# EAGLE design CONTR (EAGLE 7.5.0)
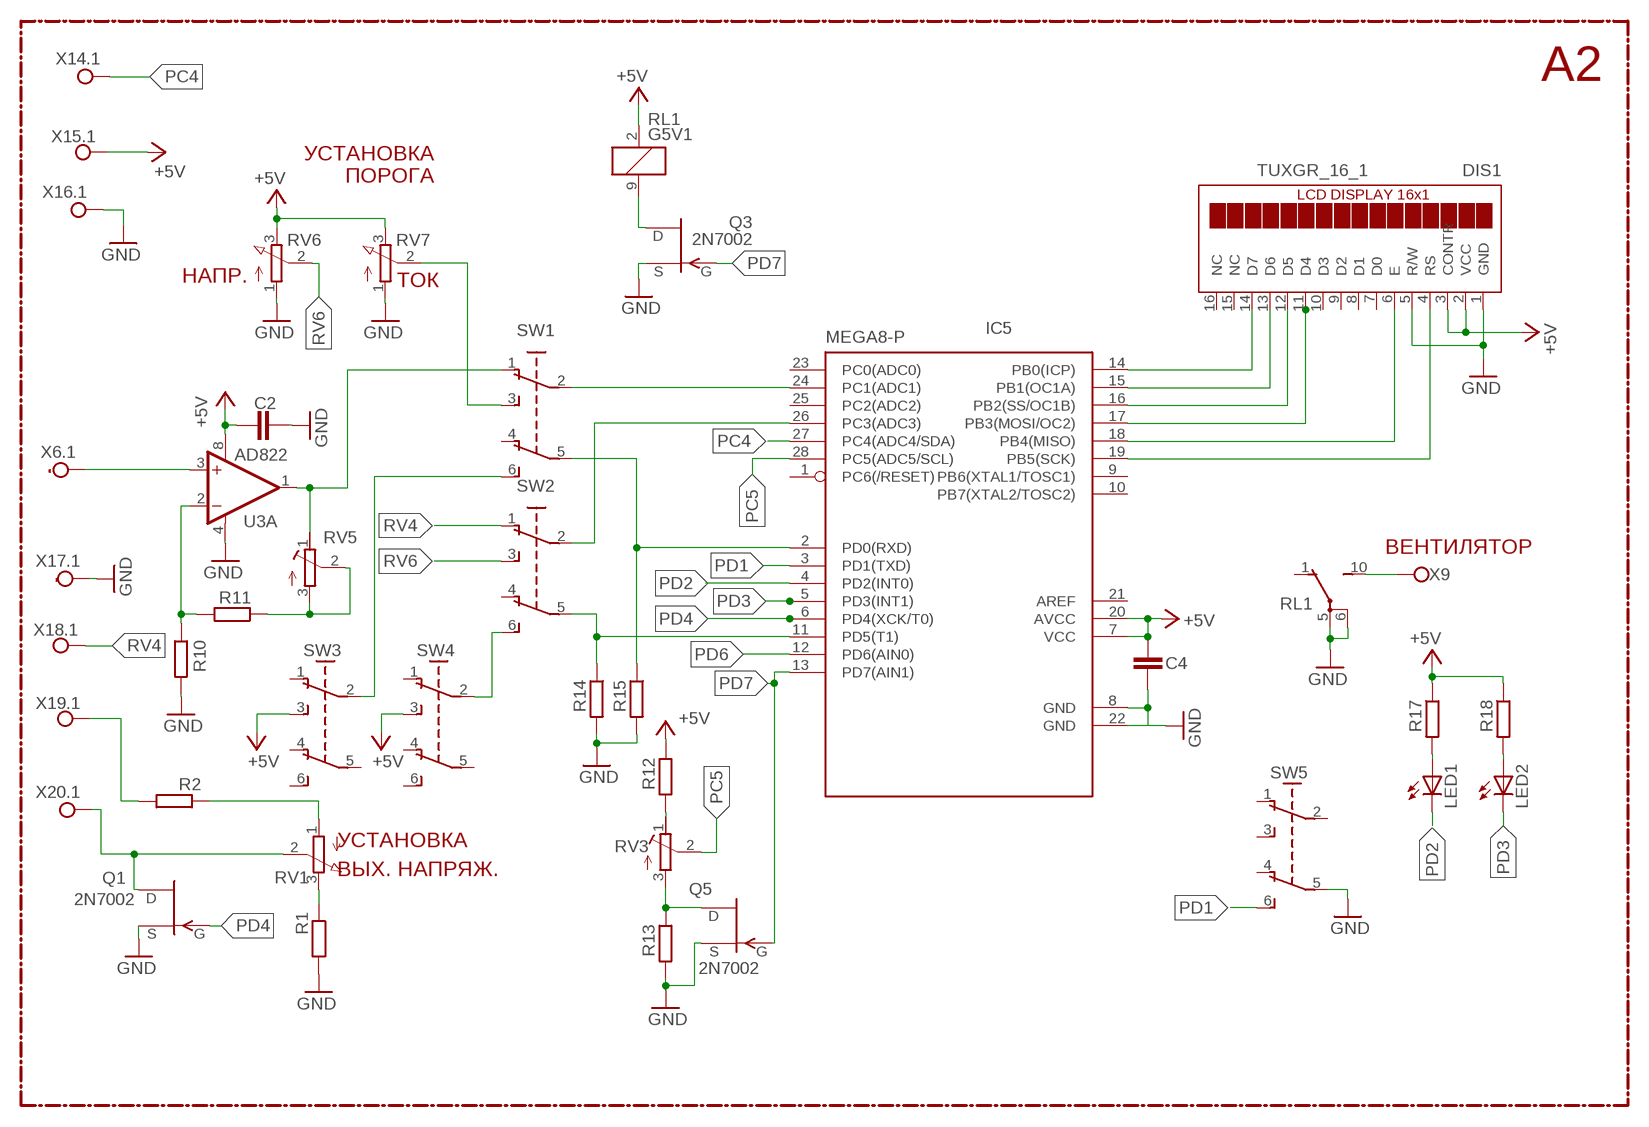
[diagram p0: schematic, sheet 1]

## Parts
C2  C-EUC1206  [C1206]
C4  C-EUC1206  [C1206]
DIS1  TUXGR_16_1  [TUXGR_16X1]
IC5  MEGA8-P  [DIL28-3]
LED1  LED3MM  [LED3MM]
LED2  LED3MM  [LED3MM]
Q1  2N7002  SST201  [SOT23]
Q3  2N7002  SST201  [SOT23]
Q5  2N7002  SST201  [SOT23]
R1  R-EU_R1206  [R1206]
R2  R-EU_R1206  [R1206]
R10  R-EU_R1206  [R1206]
R11  R-EU_R1206  [R1206]
R12  R-EU_R1206  [R1206]
R13  R-EU_R1206  [R1206]
R14  R-EU_R1206  [R1206]
R15  R-EU_R1206  [R1206]
R17  R-EU_R1206  [R1206]
R18  R-EU_R1206  [R1206]
RL1  G5V1  [G5V1]
RV1  PTV09A  PV09A  [PTV09]
RV3  R-TRIMM-3386-F  [R-TRIMM-3386F]
RV5  R-TRIMM-3386-F  [R-TRIMM-3386F]
RV6  PTV09A  PV09A  [PTV09]
RV7  PTV09A  PV09A  [PTV09]
SW1  ESB30B102  [ESB30B102]
SW2  ESB30B102  [ESB30B102]
SW3  ESB30B102  [ESB30B102]
SW4  ESB30B102  [ESB30B102]
SW5  ESB30B102  [ESB30B102]
U3  AD822  OPA2134P  [DIL08]
X6.1  TPPAD1-20  [P1-20]
X9  TPPAD1-20  [P1-20]
X14.1  TPPAD1-20  [P1-20]
X15.1  TPPAD1-20  [P1-20]
X16.1  TPPAD1-20  [P1-20]
X17.1  TPPAD1-20  [P1-20]
X18.1  TPPAD1-20  [P1-20]
X19.1  TPPAD1-20  [P1-20]
X20.1  TPPAD1-20  [P1-20]

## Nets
+5V: C2.2 C4.2 DIS1.2(VCC) DIS1.3(CONTR) IC5.7(VCC) IC5.20(AVCC) R12.1 R17.1 R18.1 RL1.2 RV6.3(E) RV7.3(E) SW3.3 SW4.3 U3.8(A:V+) X15.1.TP
GND: C2.1 C4.1 DIS1.1(GND) DIS1.5(R/W) IC5.8(GND) IC5.22(GND) Q1.2(S) Q3.2(S) Q5.2(S) R1.2 R10.2 R13.2 R14.2 R15.2 RL1.5(2:P) RL1.6(2:P) RV6.1(A) RV7.1(A) SW5.5 U3.4(A:V-) X16.1.TP X17.1.TP
N$2: R2.1 RV1.1(A)
N$3: Q1.1(D) RV1.2(S) X20.1.TP
N$4: R1.1 RV1.3(E)
N$8: U3.3(A:+IN) X6.1.TP
N$14: DIS1.14(D7) IC5.14(PB0(ICP))
N$15: DIS1.13(D6) IC5.15(PB1(OC1A))
N$16: DIS1.12(D5) IC5.16(PB2(SS/OC1B))
N$17: DIS1.11(D4) IC5.17(PB3(MOSI/OC2))
N$18: DIS1.6(E) IC5.18(PB4(MISO))
N$19: DIS1.4(RS) IC5.19(PB5(SCK))
N$20: R10.1 R11.2 U3.2(A:-IN)
N$21: R11.1 RV5.2(S) RV5.3(E)
N$22: IC5.24(PC1(ADC1)) SW1.2
N$23: RV7.2(S) SW1.3
N$24: RV5.1(A) SW1.1 U3.1(A:OUT)
N$25: Q3.1(D) RL1.9
N$26: SW1.6 SW3.2
N$27: IC5.26(PC3(ADC3)) SW2.2
N$29: IC5.11(PD5(T1)) R14.1 SW2.5
N$30: SW2.6 SW4.2
N$31: IC5.2(PD0(RXD)) R15.1 SW1.5
N$32: RL1.10(2:S) X9.TP
N$35: R12.2 RV3.1(A)
N$36: Q5.1(D) R13.1 RV3.3(E)
N$39: R2.2 X19.1.TP
N$40: LED2.A R18.2
N$41: LED1.A R17.2
PC4: IC5.27(PC4(ADC4/SDA)) X14.1.TP
PC5: IC5.28(PC5(ADC5/SCL)) RV3.2(S)
PD1: IC5.3(PD1(TXD)) SW5.6
PD2: IC5.4(PD2(INT0)) LED1.K(C)
PD3: IC5.5(PD3(INT1)) LED2.K(C)
PD4: IC5.6(PD4(XCK/T0)) Q1.3(G)
PD6: IC5.12(PD6(AIN0))
PD7: IC5.13(PD7(AIN1)) Q3.3(G) Q5.3(G)
RV4: SW2.1 X18.1.TP
RV6: RV6.2(S) SW2.3
Unconnected: DIS1.7(D0) DIS1.8(D1) DIS1.9(D2) DIS1.10(D3) DIS1.15(NC) DIS1.16(NC) IC5.1(PC6(/RESET)) IC5.9(PB6(XTAL1/TOSC1)) IC5.10(PB7(XTAL2/TOSC2)) IC5.21(AREF) IC5.23(PC0(ADC0)) IC5.25(PC2(ADC2)) RL1.1(2:O) SW1.4 SW2.4 SW3.1 SW3.4 SW3.5 SW3.6 SW4.1 SW4.4 SW4.5 SW4.6 SW5.1 SW5.2 SW5.3 SW5.4 U3.5(B:+IN) U3.6(B:-IN) U3.7(B:OUT)

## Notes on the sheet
- A2
- УСТАНОВКА
- ПОРОГА
- НАПР. | ТОК
- ВЕНТИЛЯТОР
- УСТАНОВКА
- ВЫХ. НАПРЯЖ.

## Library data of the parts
C2 C4 = rcl:C-EU: CAPACITOR, European symbol
DIS1 = display-lcd:TUXGR_16_1: 1x16 LCD DISPLAY
IC5 = atmel:MEGA8-P: MICROCONTROLLER 8 Kbytes FLASH, 1 kbytes SRAM, 512 bytes EEPROM, USART, 4-channel 10 bit ADC, 2-channel 8 bit ADC Pin compatible with Atmega48, ATMega88, ATMega168 Source: avr.lbr; OC_FARNELL: unknown; OC_NEWARK: unknown
LED1 LED2 = led:LED: LED
Q1 Q3 Q5 = transistor-fet:?20*: TEMIC / Siliconix N-Channel JFET Source: JFET-J201_Siliconix_data.pdf
R1 R2 R10-R15 R17 R18 = rcl:R-EU_: RESISTOR, European symbol
RL1 = relay:G5V1: RELAY 1 x switch, 0.5 A/125 V AC, 1 A/24 V DC , Omron; MPN: G5V-1-DC24; OC_FARNELL: 9949593; OC_NEWARK: 36M6377
RV1 RV6 RV7 = pot:PV09A
RV3 RV5 = rcl:R-TRIMM-3386-F
SW1-SW5 = switch:ESB30B102
U3 = burr-brown:OPA2134: Operational Amplifier; MF: TEXAS INSTRUMENTS; MPN: OPA2134PA; OC_FARNELL: 1097574; OC_NEWARK: 74K3897
X6.1 X9 X14.1 X15.1 X16.1 X17.1 X18.1 X19.1 X20.1 = testpad:TP: Test pad

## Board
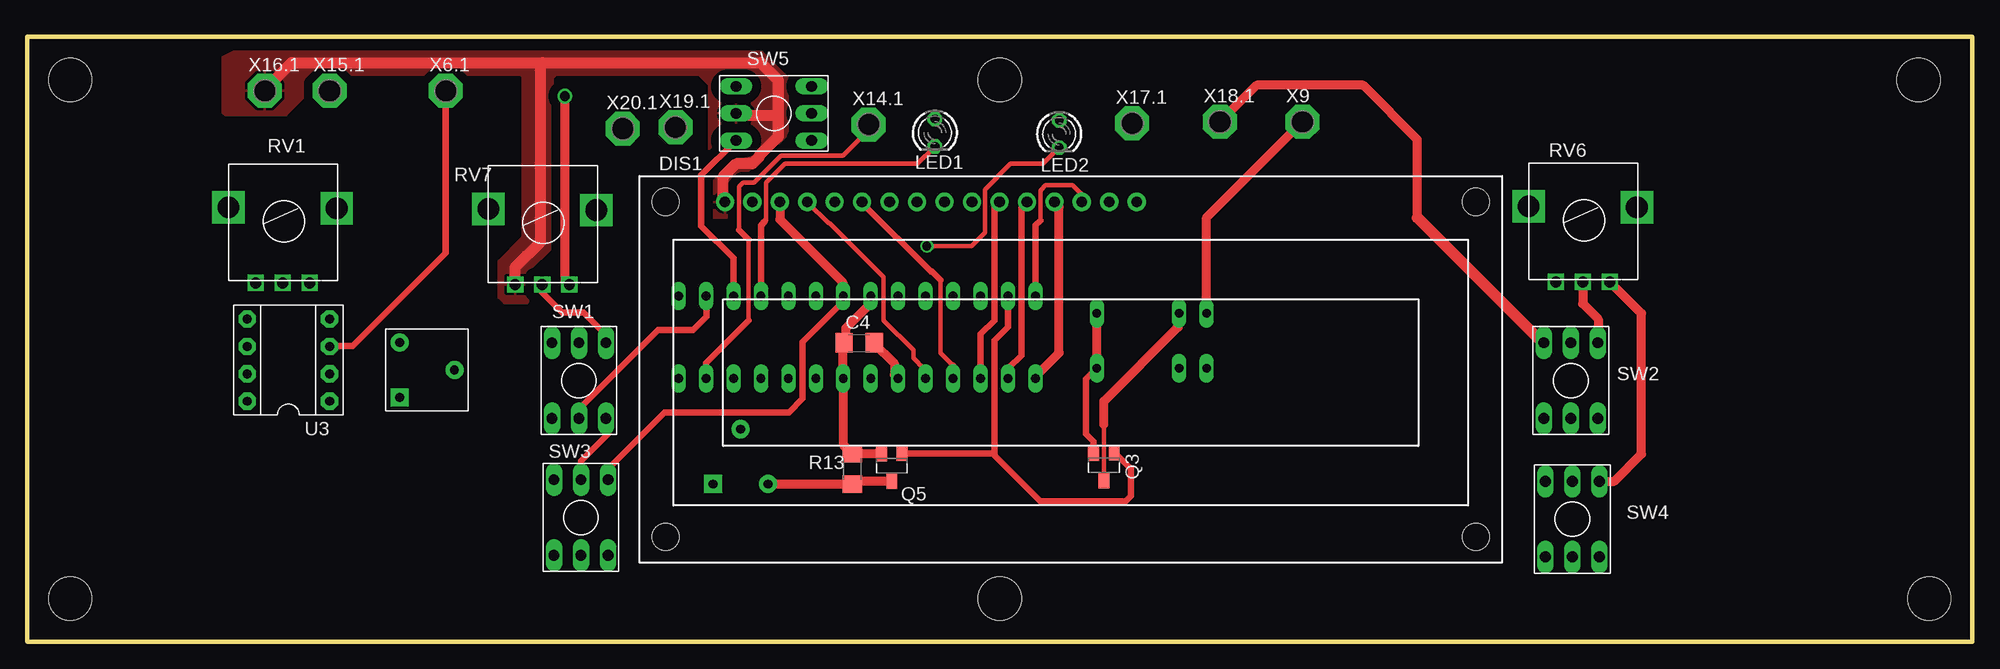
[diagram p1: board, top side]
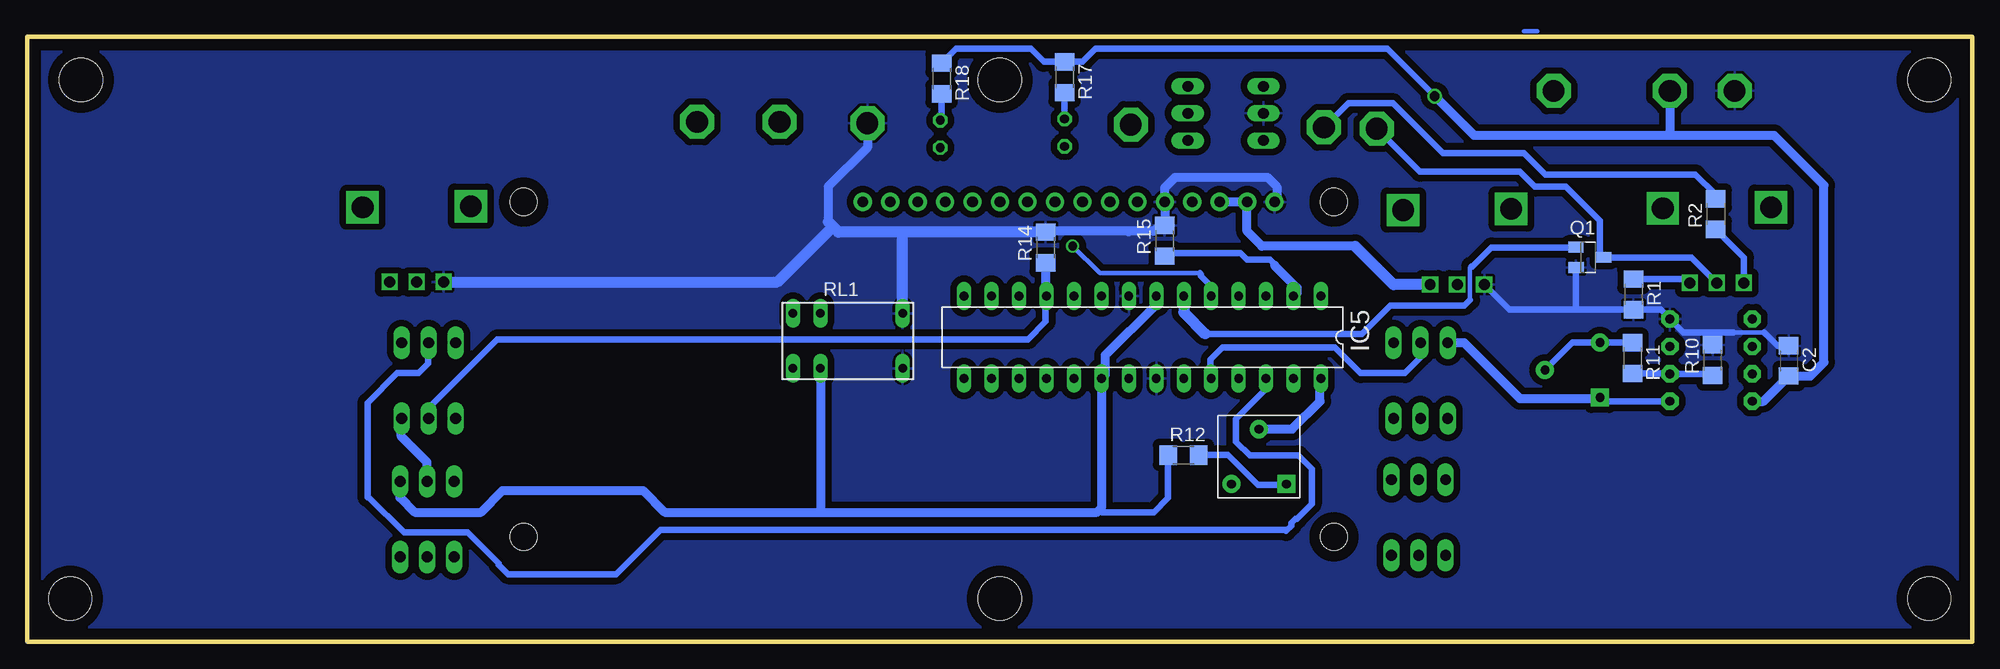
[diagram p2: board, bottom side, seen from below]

Size 180 x 56 mm. Coordinates in mm from the lower left corner, seen from the top.
Outline: 0,0 160,0
Outline: 0,0 0,56 180,56 180,0 0,0
Copper layers (1*16): Top 0.035mm / dielectric 1.5mm / Bottom 0.035mm
Design rules "default": minimum track width 10mil, minimum drill 24mil, track to track 8mil, track to pad 8mil, pad to pad 8mil, via to via 8mil, smd to smd 8mil, copper to edge 40mil, drill to drill 8mil, minimum pad ring 10mil, minimum via ring 8mil, stop-mask expansion 4mil, vias tented up to drill 0mil, thermal gap 10mil
Holes 4 mm at 4,52 4,4 90,52 90,4 175,52 176,4

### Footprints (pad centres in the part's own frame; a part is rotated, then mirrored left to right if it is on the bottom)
C1206 = smd 1.6 x 1.8: 1 -1.4,0; 2 1.4,0
TUXGR_16X1 = drill 1 pad 1.676: 1 -0.25,0.26; 2 2.29,0.26; 3 4.83,0.26; 4 7.37,0.26; 5 9.91,0.26; 6 12.45,0.26; 7 14.99,0.26; 8 17.53,0.26; 9 20.07,0.26; 10 22.61,0.26; 11 25.15,0.26; 12 27.69,0.26; 13 30.23,0.26; 14 32.77,0.26; 15 35.31,0.26; 16 37.85,0.26 | hole 2.5: -5.75,-30.74; 69.25,-30.74; -5.75,0.26; 69.25,0.26
DIL28-3 = drill 0.813 long: 1 -16.51,-3.81; 2 -13.97,-3.81; 3 -11.43,-3.81; 4 -8.89,-3.81; 5 -6.35,-3.81; 6 -3.81,-3.81; 7 -1.27,-3.81; 8 1.27,-3.81; 9 3.81,-3.81; 10 6.35,-3.81; 11 8.89,-3.81; 12 11.43,-3.81; 13 13.97,-3.81; 14 16.51,-3.81; 15 16.51,3.81; 16 13.97,3.81; 17 11.43,3.81; 18 8.89,3.81; 19 6.35,3.81; 20 3.81,3.81; 21 1.27,3.81; 22 -1.27,3.81; 23 -3.81,3.81; 24 -6.35,3.81; 25 -8.89,3.81; 26 -11.43,3.81; 27 -13.97,3.81; 28 -16.51,3.81
LED3MM = drill 0.813 octagon: A -1.27,0; K 1.27,0
SOT23 = smd 1 x 1.4: 1 0.003,1.44; 2 0.95,-1.1; 3 -0.953,-1.123
R1206 = smd 1.6 x 1.803: 1 -1.422,0; 2 1.422,0
G5V1 = drill 0.813 long: 1 -5.08,-2.54; 2 -2.54,-2.54; 5 5.08,-2.54; 6 5.08,2.54; 9 -2.54,2.54; 10 -5.08,2.54
PTV09 = drill 1 square: 1 -2.5,0; 2 0,0; 3 2.5,0 | drill 2 square: P$4 -5,7; P$5 5,6.9
R-TRIMM-3386F = drill 0.8 pad 1.676 square: 1 0,0 | drill 0.8 pad 1.676: 2 5.08,2.54; 3 0,5.08
ESB30B102 = drill 1 long: 1 0,0; 2 2.5,0; 3 5,0; 4 0,-7; 5 2.5,-7; 6 5,-7
DIL08 = drill 0.813 pad 1.6 octagon: 1 -3.81,-3.81; 2 -1.27,-3.81; 3 1.27,-3.81; 4 3.81,-3.81; 5 3.81,3.81; 6 1.27,3.81; 7 -1.27,3.81; 8 -3.81,3.81
P1-20 = drill 2.007 pad 3.15 octagon: TP 0,0

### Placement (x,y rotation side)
C2  17,26 270 bottom
C4  76.99,27.67 0 top
DIS1  64.82,40.46 0 top
IC5  76.79,28.19 180 bottom
LED1  84,47.12 270 top
LED2  95.5,47 270 top
Q1  35.58,35.59 270 bottom
Q3  99.64,16.35 180 top
Q5  80,16.3 180 top
R1  31.36,32.16 270 bottom
R2  23.75,39.59 90 bottom
R10  24.04,26.07 90 bottom
R11  31.46,26.26 270 bottom
R12  73,17.27 0 bottom
R13  76.38,16 90 top
R14  85.75,36.5 90 bottom
R15  74.75,37.12 90 bottom
R17  84,52.25 270 bottom
R18  95.38,52.12 270 bottom
RL1  104.06,27.86 0 bottom
RV1  23.65,33.22 0 top
RV3  63.48,14.6 90 bottom
RV5  34.47,22.62 0 top
RV6  143.95,33.31 0 top
RV7  47.67,33.06 0 top
SW1  48.56,27.68 0 top
SW2  140.34,27.68 0 top
SW3  48.75,15 0 top
SW4  140.48,14.85 0 top
SW5  72.6,51.41 270 top
U3  24.18,26.07 90 top
X6.1  38.75,51 0 top
X9  118,48.12 0 top
X14.1  77.88,47.88 0 top
X15.1  28,51 0 top
X16.1  22,51 0 top
X17.1  102.25,48 0 top
X18.1  110.38,48.12 0 top
X19.1  60,47.62 0 top
X20.1  55.12,47.5 0 top

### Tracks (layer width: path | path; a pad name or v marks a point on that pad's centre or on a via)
+5V  (via drill 0.9)
  Top 0.61: SW3.3 53.75,16 59,21.25 70.5,21.25 71.75,22.5 71.75,27.73 75.52,31.5 IC5.7
  Top 0.813: DIS1.3 69.65,39.1 75.5,33.25 75.5,32.02 IC5.7 | C4.2 78.33,27.67 80.25,25.75 80.25,24.73 IC5.20 | SW4.3 146.85,14.85 149.38,17.38 149.38,30.39 RV6.3 | v49.75,50.5 49.75,33.48 RV7.3
  Bottom 0.61: R12.1 74.43,13.32 75.75,12 80.5,12 80.75,12.25 | 67.12,40.7 DIS1.2 | R18.1 94.05,54.88 87.12,54.88 85.92,53.67 R17.1 82.33,53.67 81.12,54.88 54.12,54.88 v49.75,50.5
  Bottom 0.813: IC5.7 75.52,31.23 80.25,26.5 80.25,24.73 IC5.20 80.6,12.4 80.75,12.25 81,12 106.38,12 | SW4.3 145.48,13.36 144.12,12 138,12 136,14 123,14 121,12 106.38,12 | RL1.2 106.6,12.22 106.38,12 | 57.12,36.62 65.75,36.62 67.12,38 67.12,40.7 | U3.8 19.34,22.26 C2.2 15.03,24.6 13.75,25.88 13.75,42.25 18.38,46.88 28.12,46.88 | 28.12,46.88 46.12,46.88 v49.75,50.5 | X15.1.TP 28,47 28.12,46.88 | DIS1.2 DIS1.3
  Bottom 1.016: RV7.3 53.56,33.06 57.12,36.62
GND
  Top 0.61: Q3.2 98.69,18.57 98,19.25 98,24.34 RL1.5
  Top 0.813: IC5.8 78.06,31.31 75.75,29 75.75,27.83 C4.1 75.52,27.6 IC5.22 75.52,18.28 R13.2 76.4,17.4 Q5.2 | RL1.5 RL1.6
  Top 1.016: X16.1.TP 22,51.12 24.5,53.62 47.75,53.62 | 47.75,53.62 67.88,53.62 69.5,52 69.5,48.88 | 69.5,48.88 69.5,46.75 67.75,45 67.75,44.88 67.12,44.25 65.62,44.25 64.38,43 64.38,40.91 DIS1.1 | RV7.1 45.17,34.67 47.5,37 47.5,53.38 47.75,53.62 | 65.44,48.75 65.62,48.75 | 65.62,48.75 69.38,48.75 69.5,48.88 | SW5.5 65.6,48.77 65.62,48.75
  Bottom 0.406: 19.25,28.62 22.12,28.62
  Bottom 0.61: 36.62,30.74 R1.2 28.85,30.74 U3.4 26.73,28.62 23.88,28.62 | 36.62,30.74 42.85,30.74 RV7.1 | Q1.2 36.67,30.79 36.62,30.74 | C2.1 18.02,27.4 19.25,28.62 | 22.12,28.62 23.88,28.62 | R10.2 24.04,28.46 23.88,28.62
  Bottom 0.813: 75.38,38.38 75.75,38 78,38 | 78,38 85.67,38 R14.2 | 78.06,37.94 78,38 | X17.1.TP 102.25,45.75 105.88,42.12 105.88,38.88 | R15.2 75.38,38.38 | 75.38,38.38 74.73,39.02 DIS1.5 74.73,42.02 73.75,43 65.25,43 64.38,42.12 64.38,40.91 DIS1.1
  Bottom 1.016: R14.2 99,37.92 | 99,37.92 104.92,37.92 105.44,38.44 | 105.44,38.44 105.88,38.88 | RL1.6 98.98,37.9 99,37.92 | RV6.1 110.56,33.31 105.44,38.44
  pour Bottom (isolate 0.61): 0.75,54.75 179.38,54.75 179.38,0.62 0.75,0.62
  pour Top (isolate 0.813): 19.12,54.62 68,54.62 70.38,52.25 70.38,46.88 66.25,42.75 66.25,39.62 65.88,39.25 63.38,39.25 63.12,39.5 63.12,51.5 62.12,52.5 49,52.5 48.62,52.12 48.62,36.5 46.38,34.25 46.38,31.5 46.25,31.38 44.12,31.38 43.62,31.88 43.62,35.25 45.88,37.5 45.88,52.25 45.62,52.5 27.75,52.5 24,48.75 19,48.75 18.38,48.75 18.12,49 18.12,54.12
N$1
  Bottom 0.406: 41.5,56.5 40.25,56.5
N$2
  Bottom 0.61: RV1.1 21.15,35.57 R2.1
N$3
  Bottom 0.61: RV1.2 26.02,35.59 Q1.1 34.5,35.95 34.5,39 37.62,42.12 40.5,42.12 41.88,43.5 51.12,43.5 X20.1.TP
N$4
  Bottom 0.61: R1.1 26.51,33.58 RV1.3
N$8
  Top 0.61: X6.1.TP 38.75,36 30.12,27.38 28.62,27.38 28.5,27.25 28.08,27.25 U3.3
N$14
  Top 0.406: 93.75,39 93.75,41.75 94.25,42.25 96.75,42.25 97.5,41.5 97.5,40.81 DIS1.14
  Top 0.61: IC5.14 93.3,38.55 93.75,39
N$15
  Top 0.813: IC5.15 93.3,24.55 95.5,26.75 95.5,40.27 DIS1.13
N$16
  Top 0.61: DIS1.12 92,40.21 92,26.5 90.88,25.38 90.88,24.5 IC5.16
N$17
  Top 0.61: IC5.17 88.22,28.47 89.5,29.75 89.5,40.25 DIS1.11
N$18
  Top 0.406: 84.5,33.5 84.5,26.75 85.68,25.57
  Top 0.61: IC5.18 85.68,25.57 | DIS1.6 77.27,40.6 83.62,34.25 83.75,34.25 84.5,33.5
N$19
  Top 0.406: DIS1.4 74.16,38.75 74.25,38.75 79.25,33.75 79.25,29.75 82,27 82,26.25 83,25.25 83,24.52 IC5.19
N$20
  Bottom 0.61: R11.2 28.03,24.84 U3.2 24.19,24.8 R10.1
N$21
  Bottom 0.61: R11.1 34.45,27.68 RV5.3 37.01,27.7 RV5.2
N$22
  Bottom 0.61: SW1.2 51.06,26.32 52.5,24.88 56.62,24.88 59,27.25 69.38,27.25 70.5,26.12 70.5,24.44 IC5.24
N$23
  Top 0.61: RV7.2 47.67,32.33 49.5,30.5 51.5,30.5 53.5,28.5 53.5,27.74 SW1.3
N$24
  Bottom 0.61: U3.1 34.11,22.26 RV5.1
  Bottom 0.813: SW1.1 47.05,27.68 41.88,22.5 34.59,22.5 RV5.1
N$25
  Top 0.406: Q3.1 99.63,20.12 99.62,20.12
  Top 0.813: 99.62,20.12 99.62,22.25 106.5,29.12 106.5,30.3 RL1.9
N$26
  Top 0.61: SW3.2 51.25,16.75 53.75,19.25 53.75,20.49 SW1.6
N$27
  Bottom 0.61: IC5.26 65.36,23.39 68.12,20.62 68.12,18.5 66.88,17.25 62.38,17.25 61.12,16 61.12,12.75 62.5,11.38 62.62,11.38 63,11 63,10.75 63.5,10.25 63.62,10.38 121.38,10.38 125.5,6.25 135.5,6.25 136.38,7.12 136.38,7.25 139.25,10.12 145.12,10.12 148.38,13.38 148.5,13.38 148.5,22.12 145.75,24.88 143.75,24.88 142.88,25.75 142.88,27.64 SW2.2
N$29
  Bottom 0.61: 85.75,32.07 85.75,29.62 87.38,28 136.5,28 142.84,21.66 SW2.5
  Bottom 0.813: R14.1 85.75,32.07 IC5.11
N$30
  Bottom 0.813: SW4.2 142.98,16.61 145.38,19 145.38,20.64 SW2.6
N$31
  Top 0.61: SW1.5 51.06,21.56 58.38,28.88 61.62,28.88 62.88,30.12 62.88,31.95 IC5.2
  Bottom 0.61: 64.58,34.83 64.58,34.95 65,35.38 67.12,35.38 67.75,36 74.95,36 R15.1
  Bottom 0.813: 64.58,34.83 62.5,32.75 62.5,32.32 IC5.2
N$32
  Top 0.813: RL1.10 109.14,39.27 X9.TP
N$35
  Bottom 0.61: 63.77,14.3 RV3.1 63.58,14.5 66.12,14.5 68.9,17.27 R12.2
N$36
  Top 0.813: Q5.1 76.66,14.86 R13.1 68.58,14.58 RV3.3
N$39
  Bottom 0.61: R2.2 23.75,41.38 25.62,43.25 39.5,43.25 41.5,45.25 49,45.25 53.62,49.88 57.75,49.88 X19.1.TP
N$40
  Bottom 0.61: R18.2 95.38,48.4 LED2.A
N$41
  Bottom 0.61: R17.2 LED1.A
PC4
  Top 0.406: 66.75,29.75 66.75,37.25 | 65.88,38.12 65.88,42.12 66.25,42.5 67.25,42.5 69.75,45 75.5,45 77.88,47.38
  Top 0.61: IC5.27 62.82,25.82 66.75,29.75 | 66.75,37.25 65.88,38.12 | 77.88,47.38 X14.1.TP
PC5
  Bottom 0.813: RV3.2 62.95,19.68 60.38,22.25 60.38,24.29 IC5.28
PD1
  Top 0.61: IC5.3 65.36,35.52 62.38,38.5 62.38,43.19 SW5.6
PD2
  Top 0.406: 68.25,38.88 68.38,39 68.38,42.5 70.12,44.25 82.39,44.25 LED1.K
  Top 0.61: IC5.4 67.9,38.52 68.25,38.88
PD3  (via drill 0.8)
  Top 0.406: LED2.K 94.02,44.25 91,44.25 88.62,41.88 88.62,37.88 87.38,36.62 v83.25,36.62
  Bottom 0.406: 71.5,34.12 80.75,34.12 v83.25,36.62
  Bottom 0.61: IC5.5 70.44,32.94 71.38,33.88 71.38,34 71.5,34.12
PD4
  Bottom 0.406: 46.5,31.62 46.5,34.62 46.38,34.75
  Bottom 0.61: 71,28.5 56.5,28.5 53.88,31.12 47,31.12 46.5,31.62 | 46.38,34.75 46.25,34.75 44.5,36.5 37.38,36.5 37.25,36.38 36.87,36.38 Q1.3
  Bottom 1.016: IC5.6 72.98,30.48 71,28.5
PD7
  Top 0.61: IC5.13 90.76,29.14 89.5,27.88 89.5,17.25 | Q5.3 89.33,17.42 89.5,17.25 | Q3.3 100.65,17.47 102.12,16 102.12,13.5 101.62,13 93.75,13 89.5,17.25
RV4
  Top 0.813: 128.62,39.25 128.62,46.5 123.62,51.5 113.75,51.5 X18.1.TP
  Top 1.016: SW2.1 140.19,27.68 128.62,39.25
RV6
  Top 0.813: RV6.2 143.95,31.3 145.38,29.88 145.38,27.71 SW2.3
